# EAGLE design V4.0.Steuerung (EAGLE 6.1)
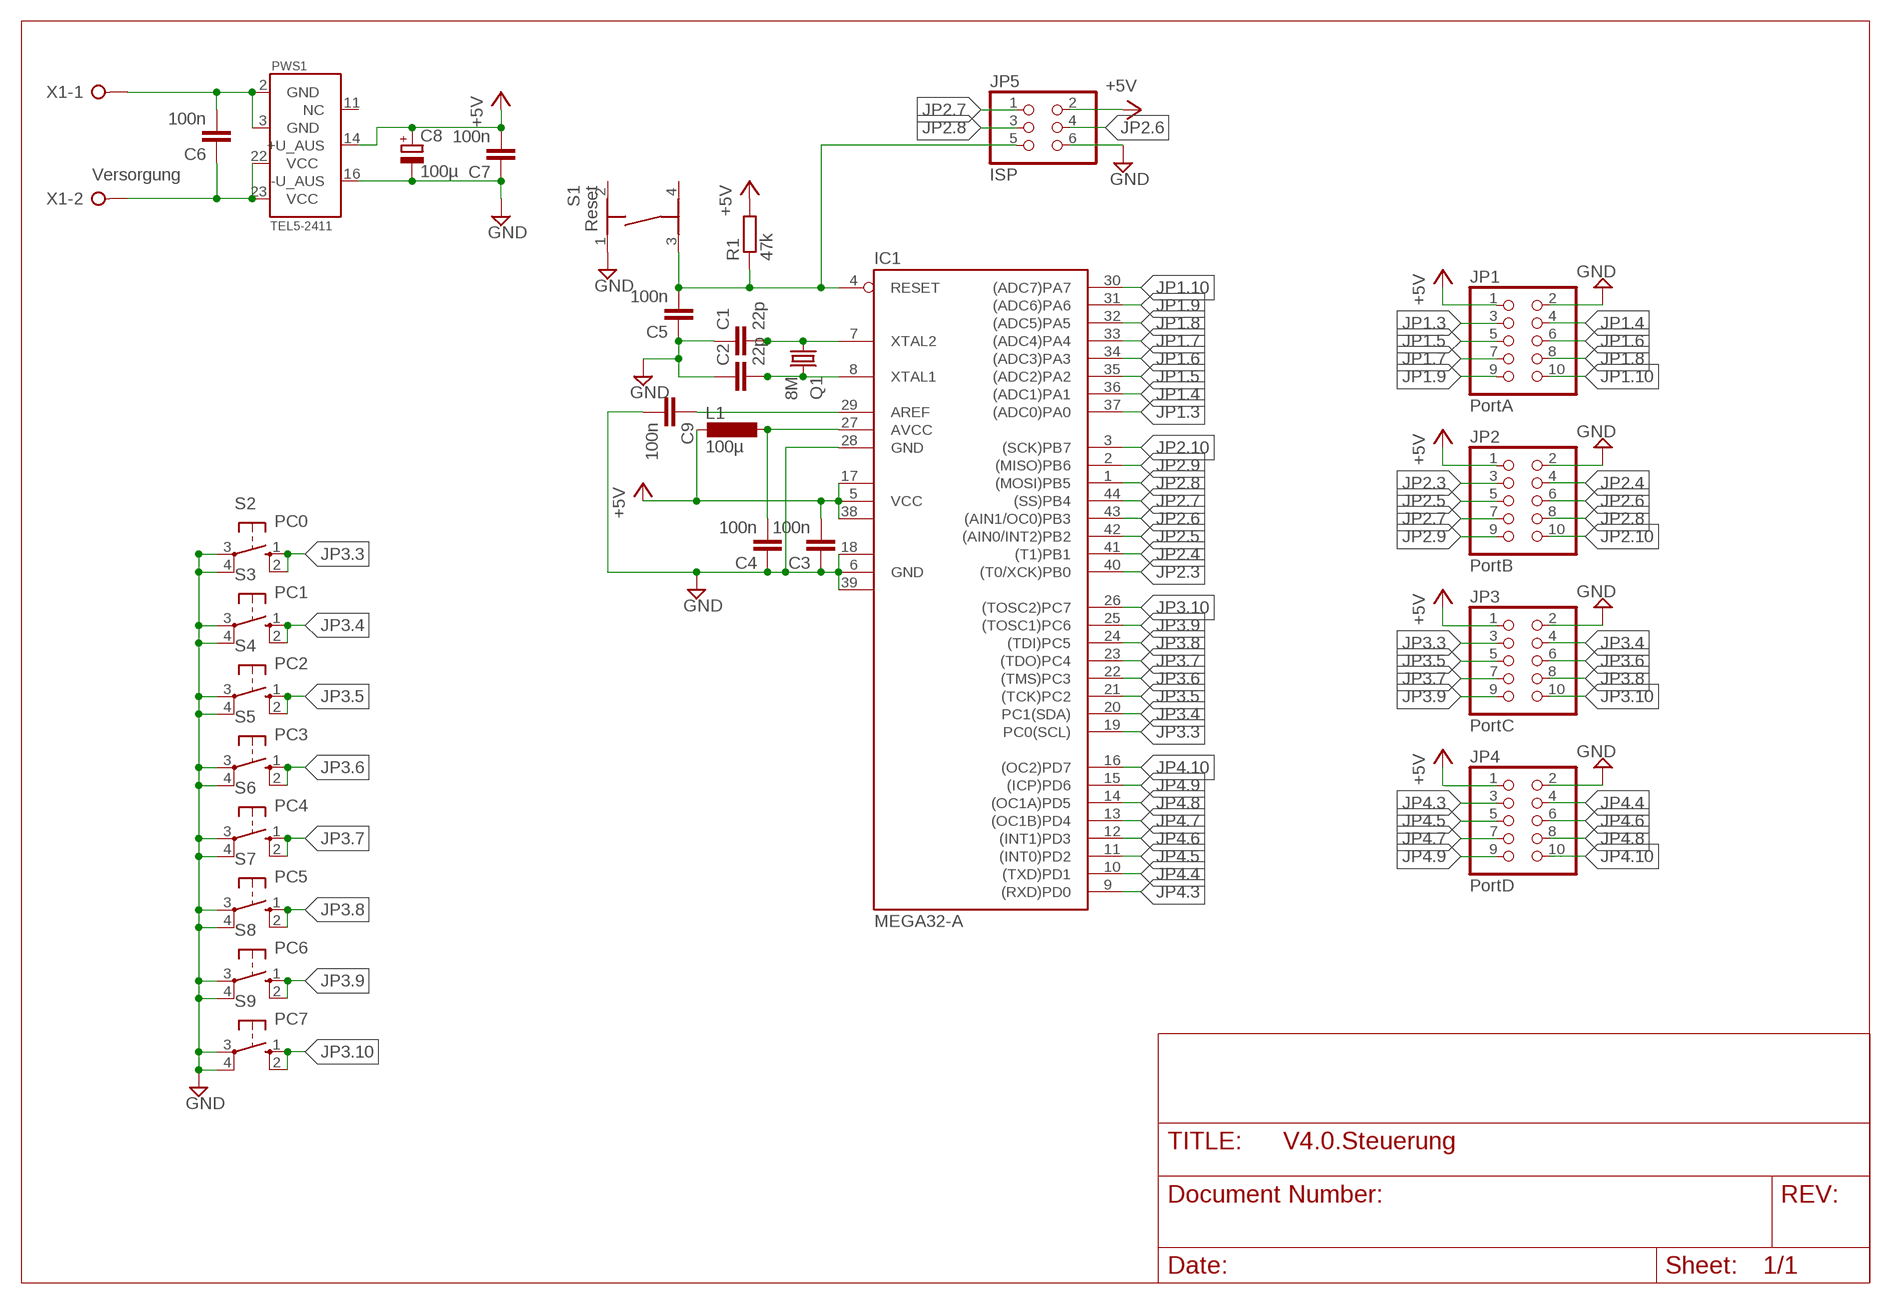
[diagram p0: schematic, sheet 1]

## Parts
C1  22p  C-EUC0402  [C0402]
C2  22p  C-EUC0402  [C0402]
C3  100n  C-EUC0402  [C0402]
C4  100n  C-EUC0402  [C0402]
C5  100n  C-EUC0402  [C0402]
C6  100n  C-EUC0402  [C0402]
C7  100n  C-EUC0402  [C0402]
C8  100µ  CPOL-EUSMCD  [SMC_D]
C9  100n  C-EUC0402  [C0402]
IC1  MEGA32-A  [TQFP44]
JP1  PortA  PINHD-2X5  [2X05]
JP2  PortB  PINHD-2X5  [2X05]
JP3  PortC  PINHD-2X5  [2X05]
JP4  PortD  PINHD-2X5  [2X05]
JP5  ISP  PINHD-2X3  [2X03]
L1  100µ  L-EUWE-TPC  [POWER-CHOKE_WE-TPC]
PWS1  TEL5-2411  [TEL5]
Q1  8M  CRYSTALHC49UP  [HC49UP]
R1  47k  R-EU_R0402  [R0402]
S1  Reset  TASTER-9314_SMD  [TASTER-9314_SMD]
S2  PC0  10-XX  [B3F-10XX]
S3  PC1  10-XX  [B3F-10XX]
S4  PC2  10-XX  [B3F-10XX]
S5  PC3  10-XX  [B3F-10XX]
S6  PC4  10-XX  [B3F-10XX]
S7  PC5  10-XX  [B3F-10XX]
S8  PC6  10-XX  [B3F-10XX]
S9  PC7  10-XX  [B3F-10XX]
X1  Versorgung  W237-02P  [W237-132]

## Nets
+5V: C3.2 C7.2 C8.+ IC1.5(VCC) IC1.17(VCC1) IC1.38(VCC2) JP1.1 JP2.1 JP3.1 JP4.1 JP5.2 L1.2 PWS1.14(+U_AUS) R1.2
GND: C1.1 C2.1 C3.1 C4.1 C5.1 C7.1 C8.- C9.2 IC1.6(GND) IC1.18(GND1) IC1.28(GND) IC1.39(GND2) JP1.2 JP2.2 JP3.2 JP4.2 JP5.6 PWS1.16(-U_AUS) S1.1 S2.3(P) S2.4(P1) S3.3(P) S3.4(P1) S4.3(P) S4.4(P1) S5.3(P) S5.4(P1) S6.3(P) S6.4(P1) S7.3(P) S7.4(P1) S8.3(P) S8.4(P1) S9.3(P) S9.4(P1)
GND@1: C6.2 PWS1.2(GND) PWS1.3(GND) X1.1
JP1.3: IC1.37((ADC0)PA0) JP1.3
JP1.4: IC1.36((ADC1)PA1) JP1.4
JP1.5: IC1.35((ADC2)PA2) JP1.5
JP1.6: IC1.34((ADC3)PA3) JP1.6
JP1.7: IC1.33((ADC4)PA4) JP1.7
JP1.8: IC1.32((ADC5)PA5) JP1.8
JP1.9: IC1.31((ADC6)PA6) JP1.9
JP1.10: IC1.30((ADC7)PA7) JP1.10
JP2.3: IC1.40((T0/XCK)PB0) JP2.3
JP2.4: IC1.41((T1)PB1) JP2.4
JP2.5: IC1.42((AIN0/INT2)PB2) JP2.5
JP2.6: IC1.43((AIN1/OC0)PB3) JP2.6 JP5.4
JP2.7: IC1.44((SS)PB4) JP2.7 JP5.1
JP2.8: IC1.1((MOSI)PB5) JP2.8 JP5.3
JP2.9: IC1.2((MISO)PB6) JP2.9
JP2.10: IC1.3((SCK)PB7) JP2.10
JP3.3: IC1.19(PC0(SCL)) JP3.3 S2.1(S) S2.2(S1)
JP3.4: IC1.20(PC1(SDA)) JP3.4 S3.1(S) S3.2(S1)
JP3.5: IC1.21((TCK)PC2) JP3.5 S4.1(S) S4.2(S1)
JP3.6: IC1.22((TMS)PC3) JP3.6 S5.1(S) S5.2(S1)
JP3.7: IC1.23((TDO)PC4) JP3.7 S6.1(S) S6.2(S1)
JP3.8: IC1.24((TDI)PC5) JP3.8 S7.1(S) S7.2(S1)
JP3.9: IC1.25((TOSC1)PC6) JP3.9 S8.1(S) S8.2(S1)
JP3.10: IC1.26((TOSC2)PC7) JP3.10 S9.1(S) S9.2(S1)
JP4.3: IC1.9((RXD)PD0) JP4.3
JP4.4: IC1.10((TXD)PD1) JP4.4
JP4.5: IC1.11((INT0)PD2) JP4.5
JP4.6: IC1.12((INT1)PD3) JP4.6
JP4.7: IC1.13((OC1B)PD4) JP4.7
JP4.8: IC1.14((OC1A)PD5) JP4.8
JP4.9: IC1.15((ICP)PD6) JP4.9
JP4.10: IC1.16((OC2)PD7) JP4.10
N$1: C2.2 IC1.8(XTAL1) Q1.2
N$2: C9.1 IC1.29(AREF)
N$3: C4.2 IC1.27(AVCC) L1.1
N$4: C6.1 PWS1.22(VCC) PWS1.23(VCC) X1.2
N$5: C1.2 IC1.7(XTAL2) Q1.1
N$6: C5.2 IC1.4(RESET) JP5.5 R1.1 S1.3
Unconnected: PWS1.11(NC) S1.2 S1.4

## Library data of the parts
C1-C7 C9 = rcl:C-EU: CAPACITOR, European symbol
C8 = rcl:CPOL-EU: POLARIZED CAPACITOR, European symbol
IC1 = atmel:MEGA32: MICROCONTROLLER 32 Kbytes FLASH 2 Kbytes SRAM 1 Kbytes EEPROM USART 8-channel 10 bit ADC Source: www.atmel.com .. doc2503.pdf; MPN: ATMEGA32-16AU; OC_FARNELL: 9171274; OC_NEWARK: 69K6677
JP1-JP4 = pinhead:PINHD-2X5: PIN HEADER
JP5 = pinhead:PINHD-2X3: PIN HEADER
L1 = rcl:L-EU: INDUCTOR, European symbol
PWS1 = Jonas_Bib_Eagle:TEL5-2411: DC/DC Converter TEL5-2411 Source: http://www.tracopower.com/datasheet_g/tel5-d.pdf Traco Power 24V -> 5V, 5W, DIL16 Package
Q1 = crystal:CRYSTAL: CRYSTAL; OC_FARNELL: unknown; OC_NEWARK: unknown
R1 = rcl:R-EU_: RESISTOR, European symbol
S1 = Ergaenzung:TASTER-9314_SMD
S2-S9 = switch-omron:10-XX: OMRON SWITCH; MPN: B3F-1000; OC_FARNELL: 176432; OC_NEWARK: 36M3542
X1 = con-wago-508:W237-02P: WAGO SREW CLAMP; OC_FARNELL: unknown; OC_NEWARK: unknown

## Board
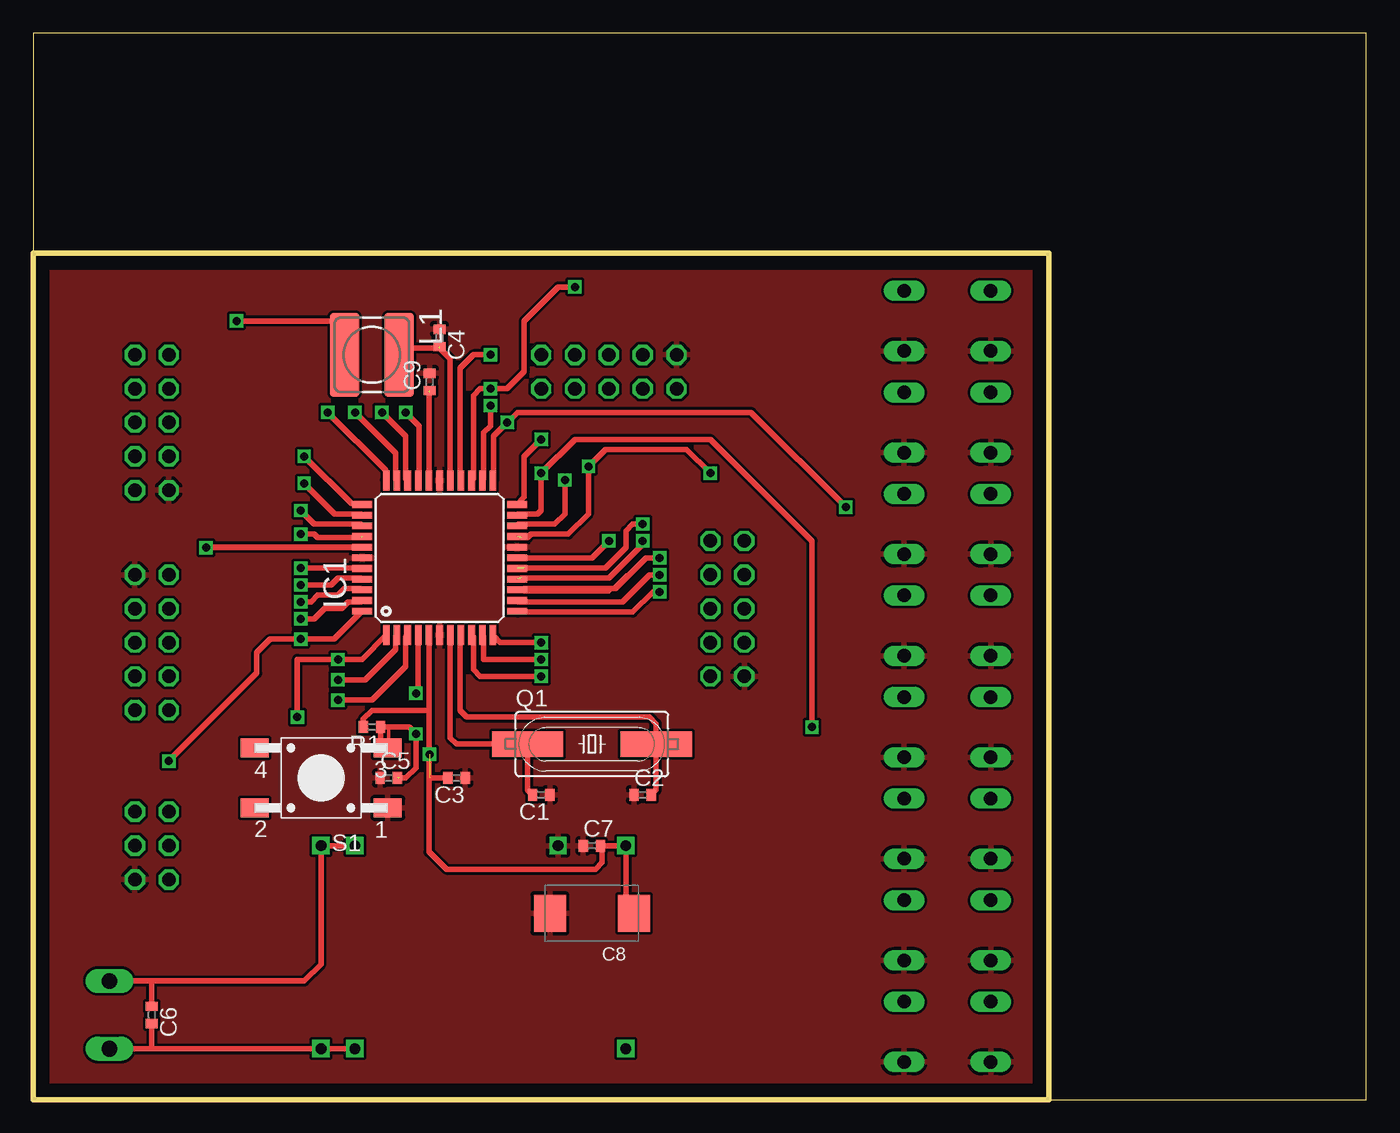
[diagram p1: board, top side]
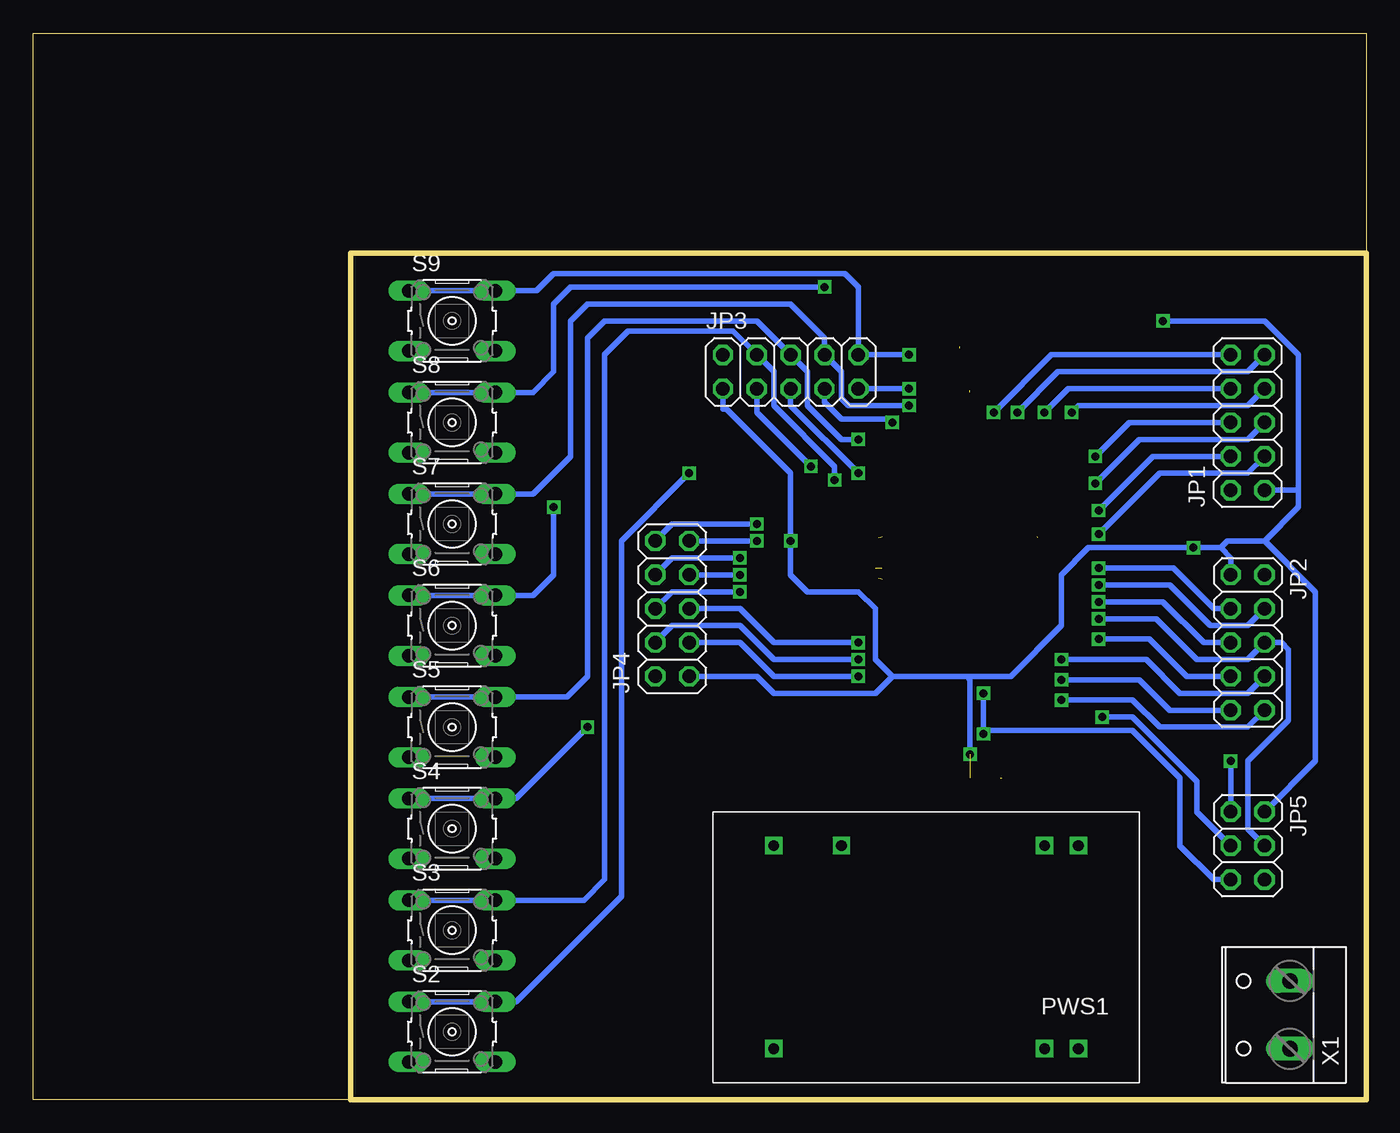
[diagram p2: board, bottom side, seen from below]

Size 100 x 80 mm. Coordinates in mm from the lower left corner, seen from the top.
Outline: 0,0 100,0 100,80 0,80 0,63.5
Outline: 0,63.5 0,0
Outline: 0,0 76.2,0 76.2,63.5 0,63.5
Copper layers (1*16): Top 0.035mm / dielectric 1.5mm / Bottom 0.035mm
Design rules: minimum track width 10mil, minimum drill 24mil, track to track 8mil, track to pad 8mil, pad to pad 8mil, via to via 8mil, smd to smd 8mil, copper to edge 40mil, drill to drill 8mil, minimum pad ring 10mil, minimum via ring 8mil, stop-mask expansion 4mil, vias tented up to drill 0mil, thermal gap 10mil

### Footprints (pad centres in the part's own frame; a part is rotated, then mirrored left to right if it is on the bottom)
C0402 = smd 0.7 x 0.9: 1 -0.65,0; 2 0.65,0
SMC_D = smd 2.4 x 2.8: + -3.15,0; - 3.15,0
TQFP44 = smd 1.5 x 0.5: 1 -5.8,4; 2 -5.8,3.2; 3 -5.8,2.4; 4 -5.8,1.6; 5 -5.8,0.8; 6 -5.8,0; 7 -5.8,-0.8; 8 -5.8,-1.6; 9 -5.8,-2.4; 10 -5.8,-3.2; 11 -5.8,-4; 23 5.8,-4; 24 5.8,-3.2; 25 5.8,-2.4; 26 5.8,-1.6; 27 5.8,-0.8; 28 5.8,0; 29 5.8,0.8; 30 5.8,1.6; 31 5.8,2.4; 32 5.8,3.2; 33 5.8,4 | smd 0.5 x 1.5: 12 -4,-5.8; 13 -3.2,-5.8; 14 -2.4,-5.8; 15 -1.6,-5.8; 16 -0.8,-5.8; 17 0,-5.8; 18 0.8,-5.8; 19 1.6,-5.8; 20 2.4,-5.8; 21 3.2,-5.8; 22 4,-5.8; 34 4,5.8; 35 3.2,5.8; 36 2.4,5.8; 37 1.6,5.8; 38 0.8,5.8; 39 0,5.8; 40 -0.8,5.8; 41 -1.6,5.8; 42 -2.4,5.8; 43 -3.2,5.8; 44 -4,5.8
2X05 = drill 1.016 octagon: 1 -5.08,-1.27; 2 -5.08,1.27; 3 -2.54,-1.27; 4 -2.54,1.27; 5 0,-1.27; 6 0,1.27; 7 2.54,-1.27; 8 2.54,1.27; 9 5.08,-1.27; 10 5.08,1.27
2X03 = drill 1.016 octagon: 1 -2.54,-1.27; 2 -2.54,1.27; 3 0,-1.27; 4 0,1.27; 5 2.54,-1.27; 6 2.54,1.27
POWER-CHOKE_WE-TPC = smd 6.3 x 2.2: 1 0,2.05; 2 0,-2.05
TEL5 = drill 0.8 square: 2 -11.43,7.62; 3 -8.89,7.62; 11 11.43,7.62; 14 11.43,-7.62; 16 6.35,-7.62; 22 -8.89,-7.62; 23 -11.43,-7.62
HC49UP = smd 5.334 x 1.93: 1 -4.826,0; 2 4.826,0
R0402 = smd 0.7 x 0.9: 1 -0.65,0; 2 0.65,0
TASTER-9314_SMD = smd 2.1 x 1.4: 1 -5,2.25; 2 5,2.25; 3 -5,-2.25; 4 5,-2.25
B3F-10XX = drill 1.016 long: 1 -3.251,2.261; 2 3.251,2.261; 3 -3.251,-2.261; 4 3.251,-2.261
W237-132 = drill 1.194 long: 1 -2.54,-0.635; 2 2.54,-0.635

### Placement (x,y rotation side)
C1  38.1,22.86 180 top
C2  45.72,22.86 0 top
C3  31.75,24.13 180 top
C4  30.48,57.15 270 top
C5  26.67,24.13 0 top
C6  8.89,6.35 270 top
C7  41.91,19.05 0 top
C8  41.91,13.97 180 top
C9  29.72,53.85 90 top
IC1  30.48,40.64 90 top
JP1  8.89,50.8 90 bottom
JP2  8.89,34.29 270 bottom
JP3  43.18,54.61 0 bottom
JP4  52.07,36.83 90 bottom
JP5  8.89,19.05 270 bottom
L1  25.4,55.88 270 top
PWS1  33.02,11.43 180 bottom
Q1  41.91,26.67 0 top
R1  25.4,27.94 180 top
S1  21.59,24.13 180 top
S2  68.58,5.08 0 bottom
S3  68.58,12.7 0 bottom
S4  68.58,20.32 0 bottom
S5  68.58,27.94 0 bottom
S6  68.58,35.56 0 bottom
S7  68.58,43.18 0 bottom
S8  68.58,50.8 0 bottom
S9  68.58,58.42 0 bottom
X1  6.35,6.35 90 bottom

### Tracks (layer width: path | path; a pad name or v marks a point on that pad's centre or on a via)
+5V  (via drill 0.6)  (1 unrouted)
  Top 0.254: 44.45,13.97 C8.+
  Top 0.406: 44.45,13.97 PWS1.14 42.67,19.05 | C7.2 42.67,19.05 | IC1.5 29.68,29.21 | 29.68,25.95 29.68,18.58 30.99,17.27 42.16,17.27 42.67,17.78 42.67,19.05 | R1.2 24.75,28.56 25.4,29.21 29.68,29.21 | C3.2 29.72,24.13 | 29.68,29.21 29.68,25.95 | 29.68,25.95 v29.72,25.91 | L1.2 23.35,56.66 22.86,57.15 22.86,58.42 v15.24,58.42 | IC1.17 41.91,40.64 v43.18,41.91 | 24.64,41.4 IC1.38 12.99,41.44 v12.95,41.4 24.64,41.4
  Bottom 0.406: 10.92,41.4 v12.95,41.4 20.83,41.4 22.86,39.37 22.86,35.56 26.67,31.75 29.97,31.75 | 10.92,41.4 10.16,40.64 JP2.1 | 5.08,45.72 5.08,55.88 7.62,58.42 v15.24,58.42 | 5.08,45.72 5.08,44.45 7.62,41.91 | 7.62,41.91 10.41,41.91 10.92,41.4 | JP1.1 5.08,45.72 | 29.97,31.75 35.56,31.75 | 35.56,31.75 36.83,33.02 36.83,36.83 38.1,38.1 41.91,38.1 43.18,39.37 v43.18,41.91 43.18,46.99 48.01,51.82 48.26,51.82 JP3.1 | v29.72,25.91 29.72,31.5 29.97,31.75 | JP4.1 45.72,31.75 44.45,30.48 36.83,30.48 35.56,31.75 | JP5.2 3.81,25.4 3.81,38.1 7.62,41.91
GND
  pour Top: 0,0 74.93,0 74.93,62.23 0,62.23
GND@1
  Top 0.406: X1.1 8.89,3.81 | 8.89,3.81 PWS1.2 PWS1.3 | C6.2 8.89,3.81
JP1.3  (via drill 0.6)  (1 unrouted)
  Top 0.406: v20.07,42.42 21.08,42.42 21.34,42.16 24.64,42.16
  Bottom 0.406: JP1.3 8.89,46.99 15.49,46.99 v20.07,42.42
JP1.4  (via drill 0.6)
  Top 0.406: v20.07,44.2 21.08,43.18 24.54,43.18 IC1.36
  Bottom 0.406: JP1.4 16,48.26 v20.07,44.2
JP1.5  (via drill 0.6)
  Top 0.406: v20.32,46.23 22.61,43.94 24.58,43.94 IC1.35
  Bottom 0.406: JP1.5 8.89,49.53 17.02,49.53 v20.32,46.23
JP1.6  (via drill 0.6)
  Top 0.406: v20.32,48.26 23.88,44.7 24.62,44.7 IC1.34
  Bottom 0.406: JP1.6 17.78,50.8 v20.32,48.26
JP1.7  (via drill 0.6)
  Top 0.406: v22.1,51.56 26.42,47.24 26.42,46.5 IC1.33
  Bottom 0.406: JP1.7 8.89,52.07 21.59,52.07 v22.1,51.56
JP1.8  (via drill 0.6)
  Top 0.406: v24.13,51.56 27.18,48.51 27.18,46.54 IC1.32
  Bottom 0.406: JP1.8 22.35,53.34 v24.13,51.56
JP1.9  (via drill 0.6)
  Top 0.406: v26.16,51.56 27.94,49.78 27.94,46.58 IC1.31
  Bottom 0.406: JP1.9 8.89,54.61 23.11,54.61 v26.16,51.56
JP1.10  (via drill 0.6)
  Top 0.406: v27.94,51.56 28.96,50.55 28.96,46.52 IC1.30
  Bottom 0.406: JP1.10 23.62,55.88 v27.94,51.56
JP2.3  (via drill 0.6)
  Top 0.406: v20.07,39.88 24.64,39.88 IC1.40
  Bottom 0.406: JP2.3 11.43,36.83 14.48,39.88 v20.07,39.88
JP2.4  (via drill 0.6)
  Top 0.406: v20.07,38.61 22.35,38.61 22.86,39.12 24.6,39.12 IC1.41
  Bottom 0.406: JP2.4 8.89,35.56 11.68,35.56 14.73,38.61 v20.07,38.61
JP2.5  (via drill 0.6)
  Top 0.406: v20.07,37.34 20.83,37.34 21.34,37.85 22.86,37.85 23.37,38.35 24.57,38.35 IC1.42
  Bottom 0.406: JP2.5 12.19,34.29 15.24,37.34 v20.07,37.34
JP2.6  (via drill 0.6)
  Top 0.406: v20.07,36.07 21.08,36.07 21.84,36.83 23.11,36.83 23.62,37.34 24.58,37.34 IC1.43
  Bottom 0.406: v20.07,36.07 15.75,36.07 12.7,33.02 8.89,33.02 JP2.6 6.35,34.29 5.84,33.78 5.84,28.45 8.89,25.4 8.89,20.32 JP5.4
JP2.7  (via drill 0.6)
  Top 0.406: IC1.44 22.58,34.54 v20.07,34.54 17.78,34.54 16.76,33.53 16.76,32 v10.16,25.4
  Bottom 0.406: JP2.7 13.46,31.75 16.26,34.54 v20.07,34.54 | JP5.1 v10.16,25.4
JP2.8  (via drill 0.6)
  Top 0.406: IC1.1 24.66,33.02 v22.86,33.02 19.81,33.02 v19.81,28.7
  Bottom 0.406: JP2.8 8.89,30.48 13.97,30.48 16.51,33.02 v22.86,33.02 | JP5.3 12.7,21.59 12.7,23.88 17.53,28.7 v19.81,28.7
JP2.9  (via drill 0.6)
  Top 0.406: v22.86,31.5 24.89,31.5 27.18,33.78 27.18,34.74 IC1.2
  Bottom 0.406: JP2.9 14.73,29.21 17.02,31.5 v22.86,31.5
JP2.10  (via drill 0.6)
  Top 0.406: v22.86,29.97 25.4,29.97 27.94,32.51 27.94,34.7 IC1.3
  Bottom 0.406: JP2.10 8.89,27.94 15.49,27.94 17.53,29.97 v22.86,29.97
JP3.3  (via drill 0.6)  (1 unrouted)
  Top 0.406: v50.8,46.99 49.02,48.77 42.93,48.77 v41.66,47.5 41.66,43.94 40.13,42.42 37.34,42.42 37.08,42.16 36.58,42.16
  Bottom 0.406: JP3.3 45.72,51.56 v41.66,47.5 | S2.1 S2.2 63.78,7.34 55.88,15.24 55.88,41.91 v50.8,46.99
JP3.4  (via drill 0.6)
  Top 0.406: IC1.20 36.42,43.18 39.12,43.18 39.88,43.94 v39.88,46.48
  Bottom 0.406: S3.1 S3.2 58.7,14.96 57.15,16.51 57.15,55.88 55.37,57.66 47.5,57.66 JP3.4 44.45,54.61 44.45,52.07 39.88,47.5 v39.88,46.48
JP3.5  (via drill 0.6)
  Top 0.406: IC1.21 36.38,43.94 37.85,43.94 38.1,44.2 v38.1,46.99 40.64,49.53 50.8,49.53 58.42,41.91 v58.42,27.94
  Bottom 0.406: JP3.5 43.18,52.07 v38.1,46.99 | S4.1 S4.2 63.78,22.58 v58.42,27.94
JP3.6  (via drill 0.6)
  Top 0.406: v38.1,49.53 36.83,48.26 36.83,45.19 IC1.22
  Bottom 0.406: v38.1,49.53 39.37,49.53 41.91,52.07 41.91,54.61 JP3.6 45.72,58.42 57.15,58.42 58.42,57.15 58.42,31.75 59.97,30.2 S5.2 S5.1
JP3.7  (via drill 0.6)
  Top 0.406: IC1.23 34.54,46.5 34.54,49.78 v35.56,50.8 36.32,51.56 53.85,51.56 v60.96,44.45
  Bottom 0.406: S6.1 S6.2 62.51,37.82 60.96,39.37 v60.96,44.45 | v35.56,50.8 35.81,51.05 39.37,51.05 40.64,52.32 JP3.7
JP3.8  (via drill 0.6)
  Top 0.406: v34.29,52.07 34.29,50.55 33.78,50.04 33.78,46.54 IC1.24
  Bottom 0.406: v34.29,52.07 38.86,52.07 39.37,52.58 39.37,54.61 JP3.8 40.64,57.15 43.18,59.69 58.42,59.69 59.69,58.42 59.69,48.26 62.51,45.44 S7.2 S7.1
JP3.9  (via drill 0.6)
  Top 0.406: IC1.25 33.02,46.58 33.02,52.83 33.53,53.34 v34.29,53.34 35.56,53.34 36.83,54.61 36.83,58.42 39.37,60.96 v40.64,60.96
  Bottom 0.406: JP3.9 v34.29,53.34 | S8.1 S8.2 62.51,53.06 60.96,54.61 60.96,59.69 59.69,60.96 v40.64,60.96
JP3.10  (via drill 0.6)
  Top 0.406: v34.29,55.88 33.02,55.88 32,54.86 32,46.52 IC1.26
  Bottom 0.406: v34.29,55.88 JP3.10 38.1,60.96 39.12,61.98 60.96,61.98 62.26,60.68 S9.2 S9.1
JP4.3  (via drill 0.6)
  Top 0.406: v38.1,31.75 33.53,31.75 33.02,32.26 33.02,34.7 IC1.9
  Bottom 0.406: JP4.3 46.99,34.29 44.45,31.75 v38.1,31.75
JP4.4  (via drill 0.6)
  Top 0.406: v38.1,33.02 33.78,33.02 33.78,34.74 IC1.10
  Bottom 0.406: JP4.4 52.07,35.56 46.99,35.56 44.45,33.02 v38.1,33.02
JP4.5  (via drill 0.6)
  Top 0.406: v38.1,34.29 35.03,34.29 IC1.11
  Bottom 0.406: JP4.5 46.99,36.83 44.45,34.29 v38.1,34.29
JP4.6  (via drill 0.6)
  Top 0.406: v46.99,38.1 46.48,38.1 44.96,36.58 36.34,36.58 IC1.12
  Bottom 0.406: JP4.6 52.07,38.1 v46.99,38.1
JP4.7  (via drill 0.6)
  Top 0.406: v46.99,39.37 46.23,39.37 44.2,37.34 36.38,37.34 IC1.13
  Bottom 0.406: JP4.7 v46.99,39.37
JP4.8  (via drill 0.6)
  Top 0.254: IC1.14 36.83,38.1 43.18,38.1 44.45,39.37 44.58,39.24
  Top 0.406: v46.99,40.64 45.97,40.64 44.58,39.24 43.69,38.35 36.83,38.35
  Bottom 0.406: JP4.8 52.07,40.64 v46.99,40.64
JP4.9  (via drill 0.6)  (1 unrouted)
  Top 0.406: v45.72,41.91 45.72,41.66 43.18,39.12 36.58,39.12
  Bottom 0.406: JP4.9 v45.72,41.91
JP4.10  (via drill 0.6)  (1 unrouted)
  Top 0.406: 36.32,39.88 IC1.16 | 36.83,39.88 42.93,39.88 44.45,41.4 44.45,42.67 44.96,43.18 v45.72,43.18
  Bottom 0.406: JP4.10 52.07,43.18 v45.72,43.18
N$1
  Top 0.406: IC1.8 32,34.84 32,29.21 32.51,28.7 46.23,28.7 46.74,28.19 Q1.2 46.74,23.23 C2.2
N$2  (1 unrouted)
  Top 0.406: IC1.29 29.68,53.05 29.72,53.09
N$3  (1 unrouted)
  Top 0.254: 27.94,55.88 L1.1
  Top 0.406: 27.43,55.37 27.94,55.88 28.45,56.39 30.48,56.39 31.28,55.59 IC1.27
N$4
  Top 0.406: X1.2 8.89,8.89 | 8.89,8.89 20.32,8.89 21.59,10.16 PWS1.23 PWS1.22 | C6.1 8.89,8.89
N$5
  Top 0.406: IC1.7 31.28,27.14 31.75,26.67 Q1.1 37.08,23.23 C1.2
N$6  (via drill 0.6)  (1 unrouted)
  Top 0.254: 26.67,27.94 26.67,26.67 S1.3
  Top 0.406: 26.42,26.42 26.05,26.78 R1.1 26.67,27.94 28.19,27.94 v28.7,27.43 28.7,24.89 27.94,24.13 27.43,24.13 | IC1.4 28.88,30.66 v28.7,30.48
  Bottom 0.406: v28.7,30.48 v28.7,27.43 28.45,27.69 17.53,27.69 13.97,24.13 13.97,19.05 11.43,16.51 JP5.5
